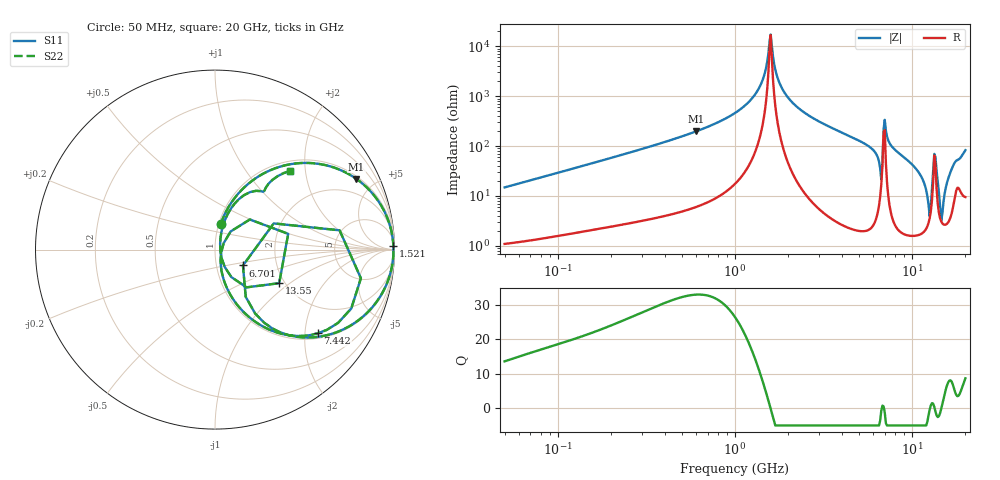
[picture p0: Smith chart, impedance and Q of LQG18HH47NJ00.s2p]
!Murata Part Number: LQG18HH47NJ00
!These Parameters are Measured in Series Mode Connection
!  o--[Z]--o
!Port1  Port2
!  o-------o
!Freq. Start=50[MHz] Stop=20[GHz], 401[Steps]
# Hz S RI R 50
!Freq.(Hz) S11(Real) S11(Imag) S21(Real) S21(Imag) S12(Real) S12(Imag) S22(Real) S22(Imag)
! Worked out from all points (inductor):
!   401 points, 50 MHz to 20 GHz, reference 50 ohm
!   read as one part in series: L = 46.8 nH near 51.52 MHz
!   highest Q = 32.9 at 600.9 MHz (marker M1), where L = 52.1 nH
!   self-resonance near 1.567 GHz
!   S11 on the Smith chart (normalised r, x): 50 MHz: 1.02, +0.30; 1.521 GHz: open; 6.701 GHz: 1.34, -0.25; 7.442 GHz: 1.14, -2.33; 13.55 GHz: 1.87, -0.84; 20 GHz: 1.19, +1.65
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5e7  0.0316 0.1418  0.9684 -0.1418  0.9684 -0.1418  0.0316 0.1418
1.364002e8  0.1475 0.3314  0.8525 -0.3314  0.8525 -0.3314  0.1475 0.3314
3.721004e8  0.5513 0.4809  0.4487 -0.4809  0.4487 -0.4809  0.5513 0.4809
6.009314e8  0.7876 0.3941  0.2124 -0.3941  0.2124 -0.3941  0.7876 0.3941
1e9  0.9482 0.2036  0.0518 -0.2036  0.0518 -0.2036  0.9482 0.2036
1.329223e9  0.9873 0.0794  0.0127 -0.0794  0.0127 -0.0794  0.9873 0.0794
1.521052e9  0.9939 0.019  0.00609 -0.019  0.00609 -0.019  0.9939 0.019
1.590961e9  0.9944 -0.00126  0.00559 0.00126  0.00559 0.00126  0.9944 -0.00126
1.875929e9  0.9889 -0.0762  0.0111 0.0762  0.0111 0.0762  0.9889 -0.0762
2.728004e9  0.9286 -0.2477  0.0714 0.2477  0.0714 0.2477  0.9286 -0.2477
5.856089e9  0.4591 -0.4862  0.5409 0.4862  0.5409 0.4862  0.4591 -0.4862
6.406762e9  0.2747 -0.4079  0.7253 0.4079  0.7253 0.4079  0.2747 -0.4079
6.701223e9  0.1557 -0.0884  0.8443 0.0884  0.8443 0.0884  0.1557 -0.0884
7.114996e9  0.759 -0.3285  0.241 0.3285  0.241 0.3285  0.759 -0.3285
7.442007e9  0.5734 -0.4664  0.4266 0.4664  0.4266 0.4664  0.5734 -0.4664
1.082228e10  0.0987 -0.2729  0.9013 0.2729  0.9013 0.2729  0.0987 -0.2729
1.238412e10  0.0312 -0.056  0.9688 0.056  0.9688 0.056  0.0312 -0.056
1.354865e10  0.3577 -0.1871  0.6423 0.1871  0.6423 0.1871  0.3577 -0.1871
1.438523e10  0.0372 -0.0486  0.9628 0.0486  0.9628 0.0486  0.0372 -0.0486
1.482269e10  0.0284 0.0319  0.9716 -0.0319  0.9716 -0.0319  0.0284 0.0319
1.670968e10  0.1338 0.2818  0.8662 -0.2818  0.8662 -0.2818  0.1338 0.2818
2e10  0.4163 0.4385  0.5837 -0.4385  0.5837 -0.4385  0.4163 0.4385
